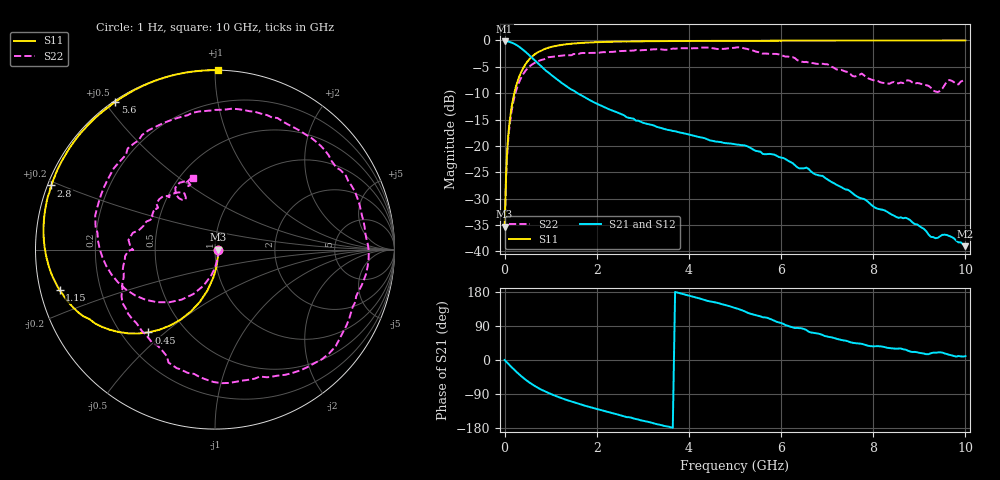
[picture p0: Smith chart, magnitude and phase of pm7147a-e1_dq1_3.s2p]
# GHz S DB R 50
! S-Parameters data
! Freq  dbS11  angS11  dbS21  angS21  dbS12  angS12  dbS22  angS22
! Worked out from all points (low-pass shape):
!   279 points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, 1 Hz to 10 GHz, reference 50 ohm
!   highest |S21| = -0.15 dB at 19.95 kHz (marker M1); lowest = -39.0 dB at 10 GHz (marker M2)
!   |S21| within 3 dB of the highest: start of sweep to 578 MHz
!   lowest |S11| = -35.3 dB at 15.85 kHz (marker M3), VSWR 1.03, Z = 51.7 - j0.00237 ohm
!   |S11| at or under -10 dB: start of sweep to 210.9 MHz
!   |S22| runs from -35.3 to -1.3 dB; largest |S21 - S12| = 0
!   S11 on the Smith chart (normalised r, x): 1 Hz: 1.03, -0.00; 450 MHz: 0.31, -0.44; 1.15 GHz: 0.06, -0.13; 2.8 GHz: 0.01, +0.19; 5.6 GHz: 0.00, +0.53; 10 GHz: 0.00, +1.02
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1e-09  -35.33 -0.0  -0.15 -0.0  -0.15 -0.0  -35.33 -0.0
1.58489e-05  -35.33 -0.1  -0.15 -0.0  -0.15 -0.0  -35.33 -0.1
1.99526e-05  -35.33 -0.1  -0.15 -0.0  -0.15 -0.0  -35.33 -0.1
0.03981072  -23.76 -78.3  -0.17 -5.0  -0.17 -5.0  -24.43 -79.1
0.1  -16.11 -93.5  -0.26 -12.5  -0.26 -12.5  -16.83 -98.2
0.25  -8.64 -111.3  -0.82 -30.5  -0.82 -30.5  -9.51 -123.7
0.45  -4.56 -128.8  -2.13 -51.5  -2.13 -51.5  -5.79 -150.3
0.75  -2.10 -148.4  -4.55 -75.2  -4.55 -75.2  -3.85 179.8
1.15  -0.97 -165.4  -7.47 -96.9  -7.47 -96.9  -2.98 150.4
1.7  -0.45 179.2  -10.58 -119.0  -10.58 -119.0  -2.37 119.1
2.8  -0.17 158.6  -14.85 -154.4  -14.85 -154.4  -1.92 66.7
3.35  -0.13 150.5  -16.50 -170.4  -16.50 -170.4  -1.67 42.0
4.3  -0.08 138.2  -18.45 160.0  -18.45 160.0  -1.34 -0.8
5.05  -0.07 129.7  -19.75 135.6  -19.75 135.6  -1.30 -38.7
5.6  -0.06 124.0  -21.50 112.8  -21.50 112.8  -2.50 -70.6
5.95  -0.05 120.5  -22.10 99.3  -22.10 99.3  -2.64 -90.6
6.7  -0.03 113.6  -25.19 71.6  -25.19 71.6  -4.31 -132.1
7.05  -0.02 110.5  -26.59 60.6  -26.59 60.6  -4.72 -153.8
7.5  -0.01 106.7  -28.59 47.0  -28.59 47.0  -6.33 -179.2
8.35  -0.00 100.1  -32.76 31.4  -32.76 31.4  -8.22 152.1
9.4  -0.00 92.8  -37.43 20.0  -37.43 20.0  -9.78 120.7
10  -0.00 89.1  -39.00 10.1  -39.00 10.1  -7.56 107.3
